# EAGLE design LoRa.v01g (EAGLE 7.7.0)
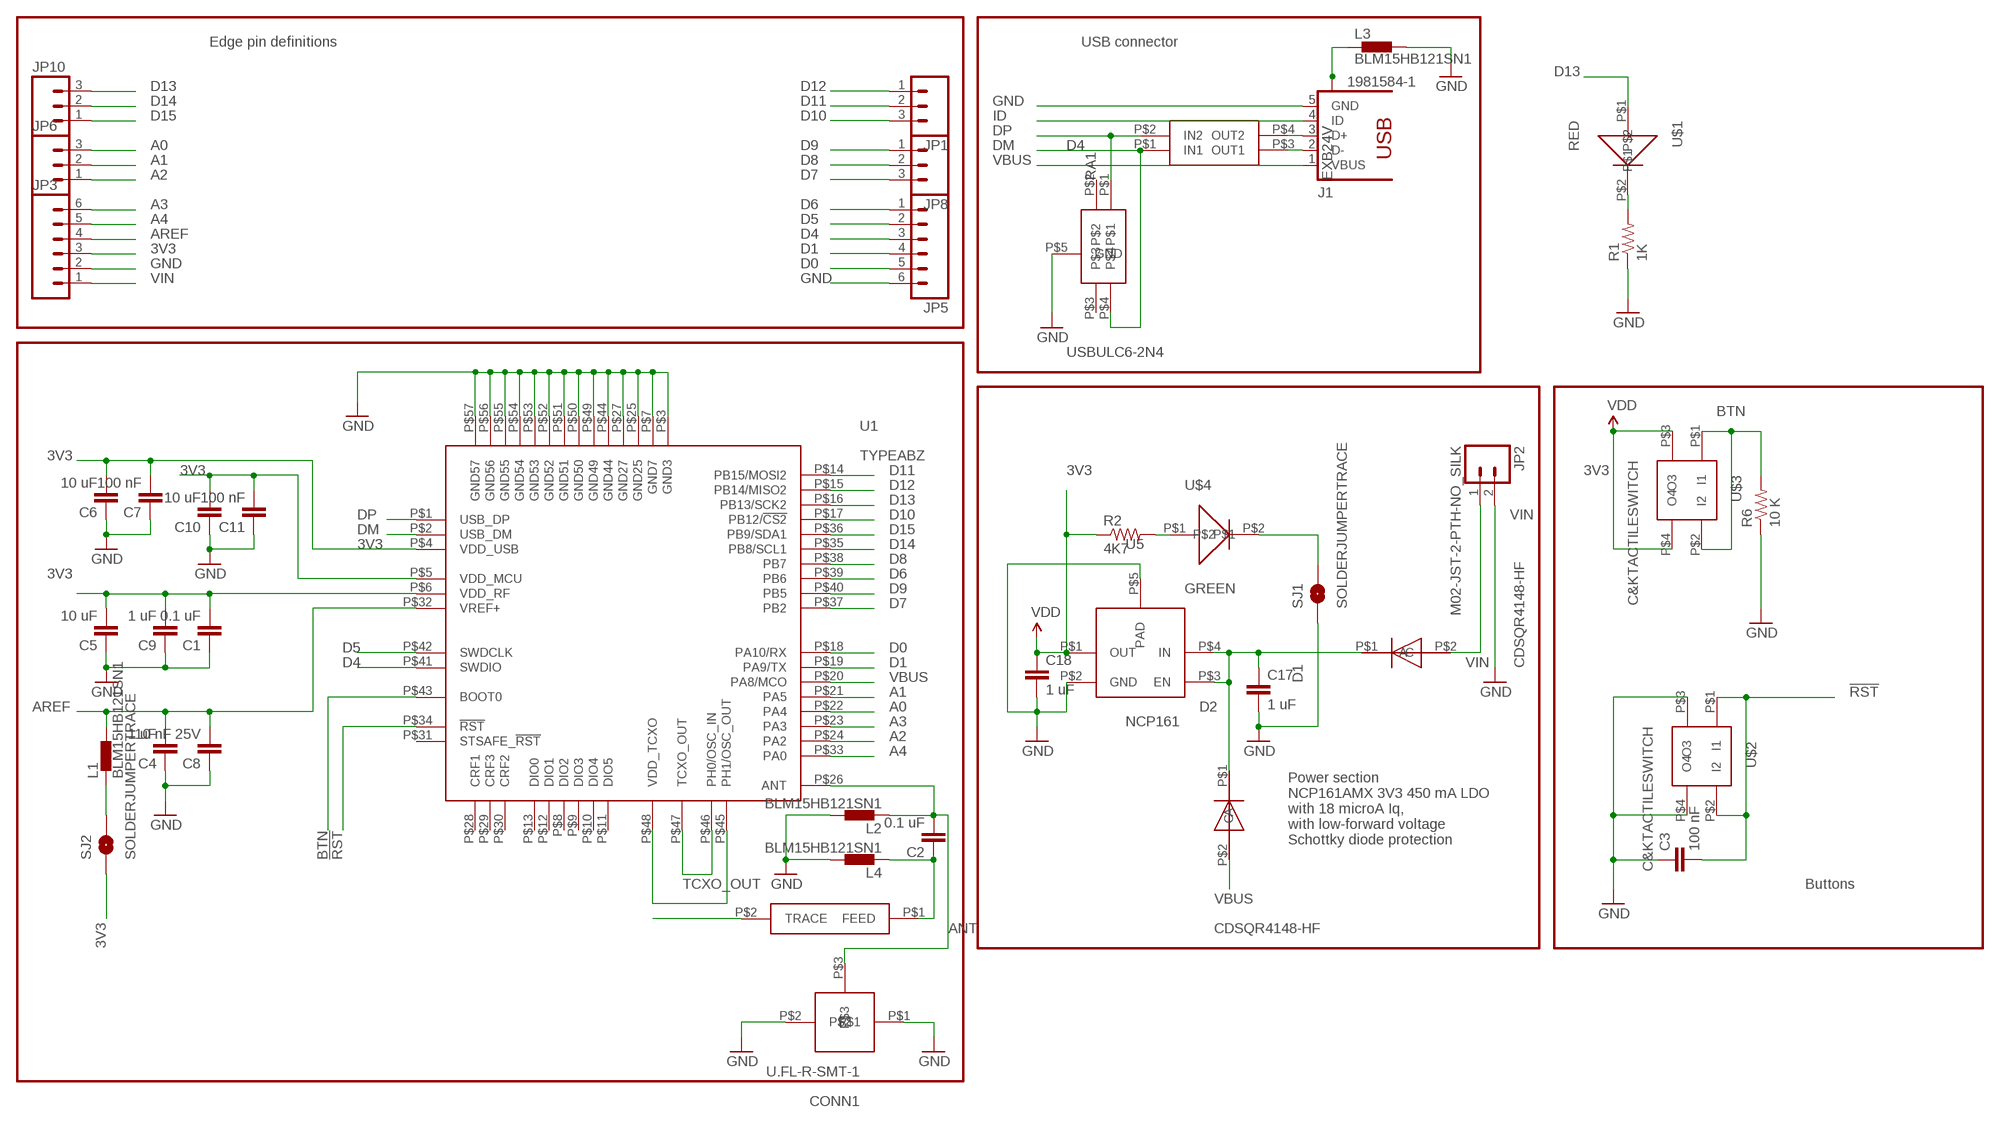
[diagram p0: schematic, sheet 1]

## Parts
C1  0.1 uF  0402CAP.KW  [0402-CAP]
C2  0.1 uF  0402CAP.KW  [0402-CAP]
C3  100 nF  0402CAP.KW  [0402-CAP]
C4  1 uF  0402CAP.KW  [0402-CAP]
C5  10 uF  0402CAP.KW  [0402-CAP]
C6  10 uF  0402CAP.KW  [0402-CAP]
C7  100 nF  0402CAP.KW  [0402-CAP]
C8  10 nF 25V  0402CAP.KW  [0402-CAP]
C9  1 uF  0402CAP.KW  [0402-CAP]
C10  10 uF  0402CAP.KW  [0402-CAP]
C11  100 nF  0402CAP.KW  [0402-CAP]
C17  1 uF  0402CAP.KW  [0402-CAP]
C18  1 uF  0402CAP.KW  [0402-CAP]
CONN1  U.FL-R-SMT-1  [U.FL-R-SMT-1]
D1  CDSQR4148-HF  [CDSQR4148-HF]
D2  CDSQR4148-HF  [CDSQR4148-HF]
D4  USBULC6-2N4  [USBULC6-2N4]
J1  1981584-1  [1981584-1]
JP1  M031X03_NO_SILK  [1X03_NO_SILK]
JP2  M02-JST-2-PTH-NO_SILK  [JST-2-PTH-NS]
JP3  M06NO_SILK  [1X06_NO_SILK]
JP5  M06NO_SILK  [1X06_NO_SILK]
JP6  M031X03_NO_SILK  [1X03_NO_SILK]
JP8  M031X03_NO_SILK  [1X03_NO_SILK]
JP10  M031X03_NO_SILK  [1X03_NO_SILK]
L1  BLM15HB121SN1  [0402]
L2  BLM15HB121SN1  [0402]
L3  BLM15HB121SN1  [0402]
L4  BLM15HB121SN1  [0402]
R1  1K  0402RES.KW  [0402-RES]
R2  4K7  0402RES.KW  [0402-RES]
R6  10 K  0402RES.KW  [0402-RES]
RA1  EXB24V  [EXB24V]
SJ1  SOLDERJUMPERTRACE  [SJ_2S-TRACE]
SJ2  SOLDERJUMPERTRACE  [SJ_2S-TRACE]
U1  TYPEABZ  [TYPEABZ]
U5  NCP161  [NCP161]
U$1  RED  0402LED  [0402LED]
U$2  C&KTACTILESWITCH  [C&KTACTILESWITCH]
U$3  C&KTACTILESWITCH  [C&KTACTILESWITCH]
U$4  GREEN  0402LED  [0402LED]
U$5  JOHANSON0900AT43A0070  [JOHANSON0900AT43A0070]

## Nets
3V3: C1.2 C5.2 C6.2 C7.2 C9.2 C10.2 C11.2 C18.1 JP3.3 R2.1 SJ2.1 U1.P$4(VDD_USB) U1.P$5(VDD_MCU) U1.P$6(VDD_RF) U5.P$1(OUT) U$3.P$3(O3) U$3.P$4(O4) ; supply symbol labelled VDD
!RST: C3.2 U1.P$34(!RST) U$2.P$1(I1) U$2.P$2(I2)
A0: JP6.3 U1.P$22(PA4)
A1: JP6.2 U1.P$21(PA5)
A2: JP6.1 U1.P$24(PA2)
A3: JP3.6 U1.P$23(PA3)
A4: JP3.5 U1.P$33(PA0)
ANT: C2.1 L4.1 U$5.P$1(FEED)
AREF: C4.2 C8.2 JP3.4 L1.2 U1.P$32(VREF+)
BTN: R6.2 U1.P$43(BOOT0) U$3.P$1(I1) U$3.P$2(I2)
D0: JP5.5 U1.P$18(PA10/RX)
D1: JP5.4 U1.P$19(PA9/TX)
D4: JP5.3 U1.P$41(SWDIO)
D5: JP5.2 U1.P$42(SWDCLK)
D6: JP5.1 U1.P$39(PB6)
D7: JP8.3 U1.P$37(PB2)
D8: JP8.2 U1.P$38(PB7)
D9: JP8.1 U1.P$40(PB5)
D10: JP1.3 U1.P$17(PB12/!CS2)
D11: JP1.2 U1.P$14(PB15/MOSI2)
D12: JP1.1 U1.P$15(PB14/MISO2)
D13: JP10.3 U1.P$16(PB13/SCK2) U$1.P$1
D14: JP10.2 U1.P$35(PB8/SCL1)
D15: JP10.1 U1.P$36(PB9/SDA1)
DM: D4.P$4 RA1.P$1(IN1) U1.P$2(USB_DM)
DP: D4.P$1 RA1.P$2(IN2) U1.P$1(USB_DP)
GND: C1.1 C3.1 C4.1 C5.1 C6.1 C7.1 C8.1 C9.1 C10.1 C11.1 C17.2 C18.2 CONN1.P$1 CONN1.P$2 D4.P$5(GND) J1.5(GND) JP2.2 JP3.2 JP5.6 L2.2 L3.2 L4.2 R1.1 R6.1 SJ1.1 U1.P$3(GND3) U1.P$7(GND7) U1.P$25(GND25) U1.P$27(GND27) U1.P$44(GND44) U1.P$49(GND49) U1.P$50(GND50) U1.P$51(GND51) U1.P$52(GND52) U1.P$53(GND53) U1.P$54(GND54) U1.P$55(GND55) U1.P$56(GND56) U1.P$57(GND57) U5.P$2(GND) U5.P$5(PAD) U$2.P$3(O3) U$2.P$4(O4)
ID: J1.4(ID)
N$1: R1.2 U$1.P$2
N$2: U$5.P$2(TRACE)
N$6: L1.1 SJ2.2
N$9: U1.P$45(PH1/OSC_OUT) U1.P$48(VDD_TCXO)
N$13: SJ1.2 U$4.P$2
N$31: J1.3(D+) RA1.P$4(OUT2)
N$32: C2.2 CONN1.P$3 L2.1 U1.P$26(ANT)
N$33: J1.2(D-) RA1.P$3(OUT1)
N$42: R2.2 U$4.P$1
N$60: C17.1 D1.P$1(C) D2.P$1(C) U5.P$3(EN) U5.P$4(IN)
TCXO_OUT: U1.P$46(PH0/OSC_IN) U1.P$47(TCXO_OUT)
USB_SHIELD: J1.S1 J1.S2 J1.S3 J1.S4 L3.1
VBUS: D2.P$2(A) J1.1(VBUS) U1.P$20(PA8/MCO)
VIN: D1.P$2(A) JP2.1 JP3.1
Unconnected: D4.P$2 D4.P$3 U1.P$8(DIO2) U1.P$9(DIO3) U1.P$10(DIO4) U1.P$11(DIO5) U1.P$12(DIO1) U1.P$13(DIO0) U1.P$28(CRF1) U1.P$29(CRF3) U1.P$30(CRF2) U1.P$31(STSAFE_!RST)

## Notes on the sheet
- Edge pin definitions | USB connector
- Power section
  NCP161AMX 3V3 450 mA LDO
  with 18 microA Iq, 
  with low-forward voltage 
  Schottky diode protection
- Buttons

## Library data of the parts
C1-C11 C17 C18 = SparkFun-Capacitors:0402CAP.KW
CONN1 = Kris:U.FL-R-SMT-1: U.FL-R-SMT-1
D1 D2 = Kris:CDSQR4148-HF: ComChip's CDSQR4148-HF high speed 150 mA Io diode
D4 = Kris:USBULC6-2N4: ST TVS diode ESD Protection USBULC6-2N4
J1 = con-usb:1981584-1: Receptacle, micro-USB, type A/B Tyco Electronics; MF: Hirose; MPN: ZX62-AB-5PA(11)
JP1 JP6 JP8 JP10 = SparkFun-Connectors:M03: Header 3 Standard 3-pin 0.1" header. Use with straight break away headers (SKU : PRT-00116), right angle break away headers (PRT-00553), swiss pins (PRT-00743), machine pins (PRT-00117), and female headers (PRT-00115). Molex polarized connector foot print use with SKU : PRT-08232 with associated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
JP2 = SparkFun-Connectors:M02: Standard 2-pin 0.1" header. Use with
JP3 JP5 = SparkFun-Connectors:M06: Header 6 Standard 6-pin 0.1" header. Use with straight break away headers (SKU : PRT-00116), right angle break away headers (PRT-00553), swiss pins (PRT-00743), machine pins (PRT-00117), and female headers (PRT-00115). Molex polarized connector foot print use with SKU : PRT-08094 with associated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
L1-L4 = inductors:BLM15H: EMIFIL (R) Chip Ferrite Bead for GHz Noise
R1 R2 R6 = SparkFun-Resistors:0402RES.KW
RA1 = Kris:EXB24V: Panasonic EXB24 22 Ohm series resistor pair
SJ1 SJ2 = SparkFun-Passives:SOLDERJUMPER: Solder Jumper
U1 = Kris:TYPEABZ: CMWX1ZZABZ-078
U5 = Kris:NCP161: NCP161 3V3 LDO voltage regulator
U$1 U$4 = Kris:0402LED: 0402led
U$2 U$3 = Kris:C&KTACTILESWITCH: C&K Tactile Switch 611-PTS810SJS250SMTR
U$5 = Kris:JOHANSON0900AT43A0070: Johanson dual wide band antenna

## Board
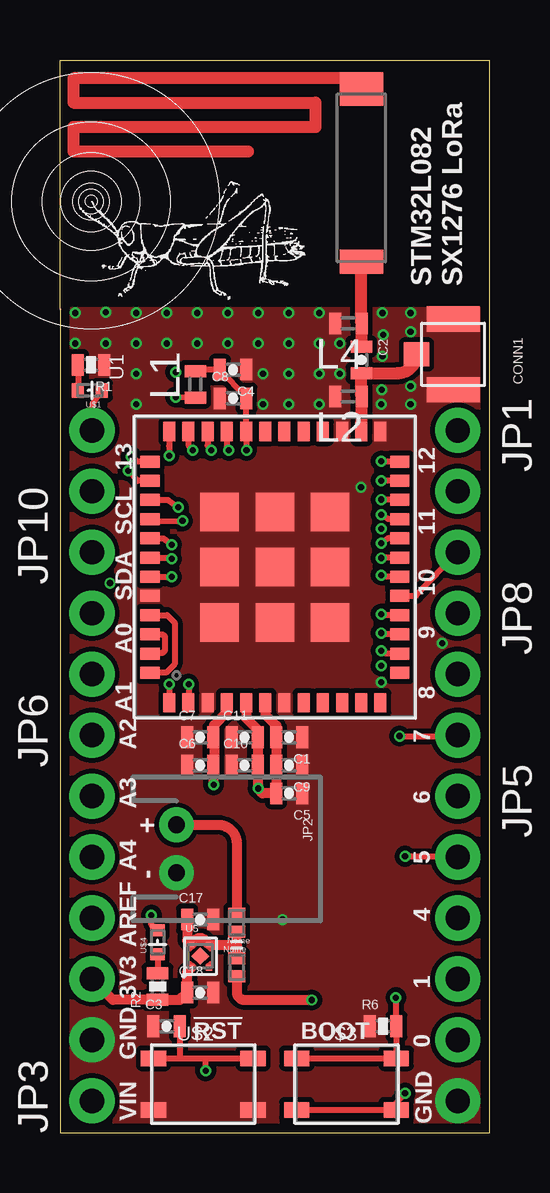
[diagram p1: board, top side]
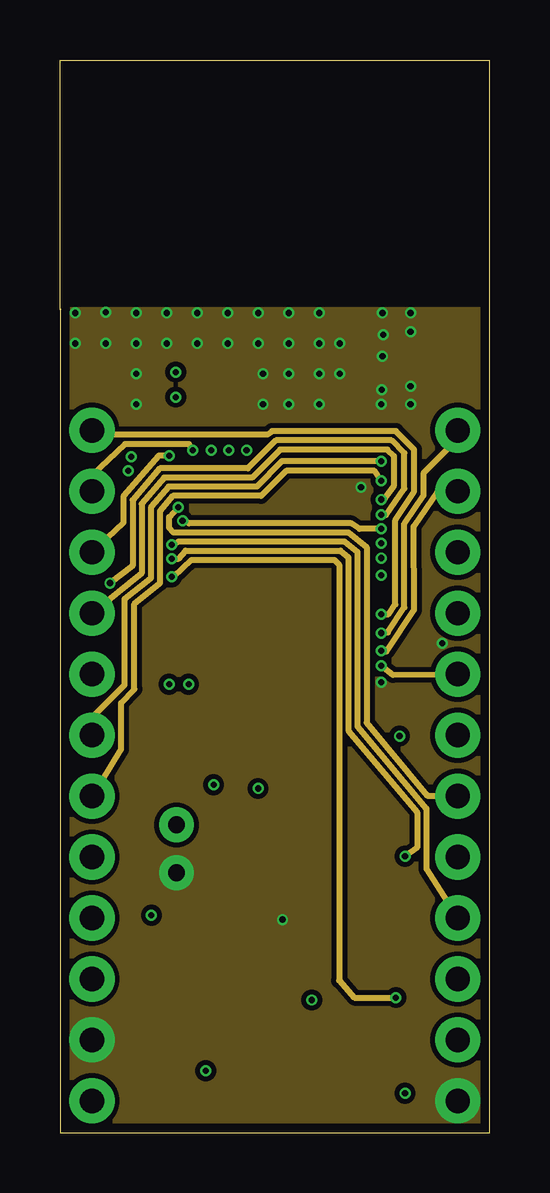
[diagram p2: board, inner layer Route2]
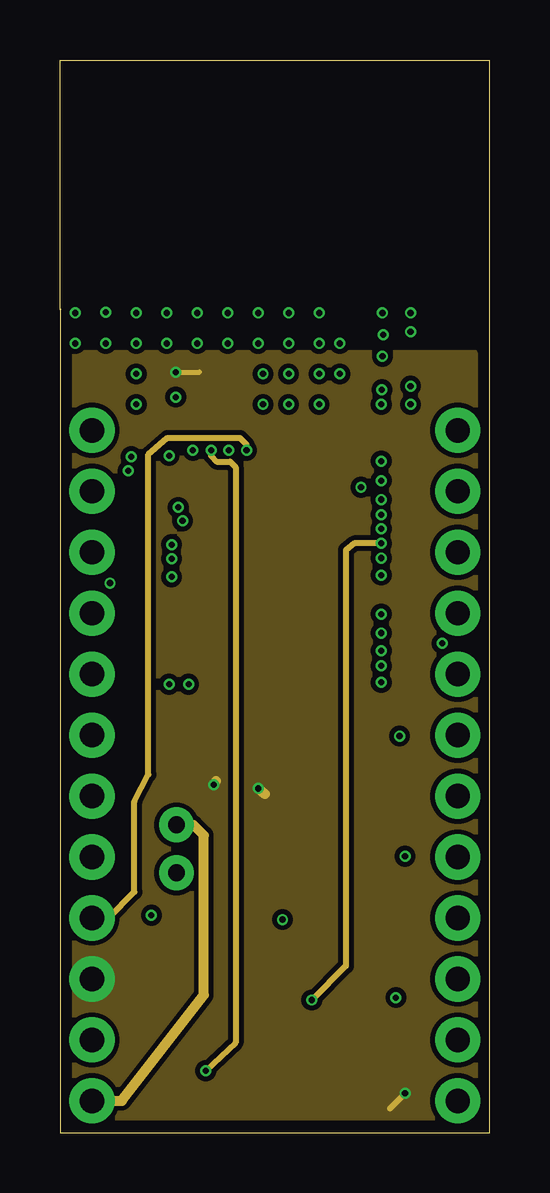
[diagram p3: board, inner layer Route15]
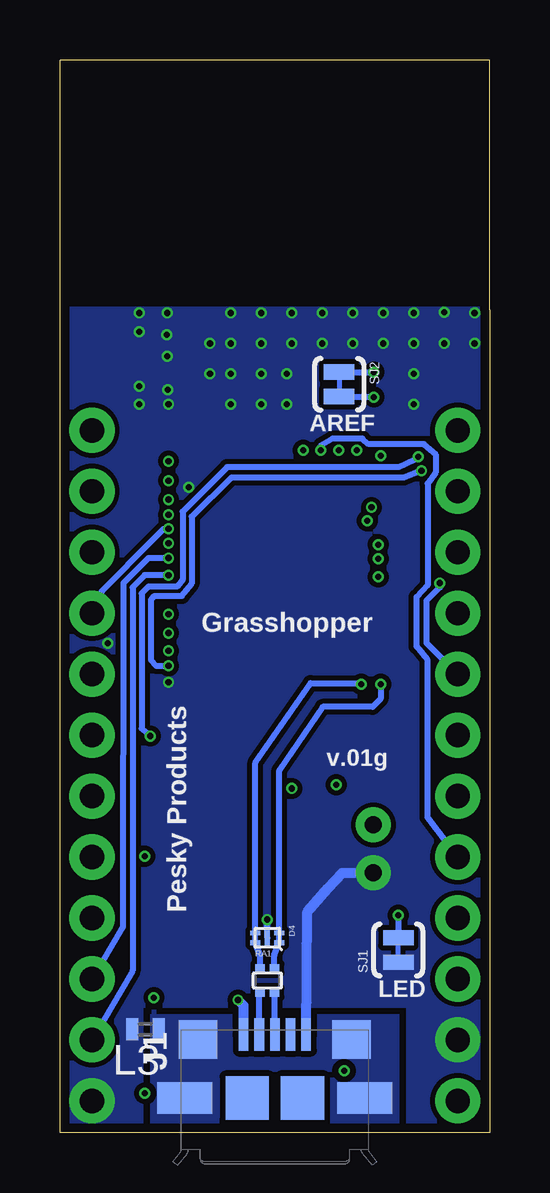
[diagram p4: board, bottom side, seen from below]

Size 17.91 x 44.7 mm. Coordinates in mm from the lower left corner, seen from the top.
Outline: 0,34.29 0,0 17.91,0 17.91,44.7 0,44.7 0,34.29
Outline: 0.03,34.31 0,34.29
Copper layers (1*2*15*16): Top 0.035559375mm / dielectric 0.17018125mm / Route2 0.01778125mm / dielectric 47mil / Route15 0.01778125mm / dielectric 0.17018125mm / Bottom 0.035559375mm
Design rules "OSHPark-4layer *": minimum track width 5mil, minimum drill 10mil, track to track 5mil, track to pad 5mil, pad to pad 5mil, via to via 5mil, smd to smd 5mil, copper to edge 15mil, drill to drill 6mil, minimum pad ring 4mil, minimum via ring 4mil, stop-mask expansion 4mil, vias tented up to drill 20mil, thermal gap 10mil

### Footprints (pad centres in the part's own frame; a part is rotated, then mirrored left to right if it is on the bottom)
0402-CAP = smd 0.5 x 0.9: 1 -0.55,0; 2 0.55,0
U.FL-R-SMT-1 = smd 1.05 x 2.2: P$1 -1.475,0; P$2 1.475,0 | smd 1 x 1.05: P$3 0,-1.525
CDSQR4148-HF = smd 0.7 x 0.5: P$1 0,0.375; P$2 0,-0.375
USBULC6-2N4 = smd 0.2 x 0.4: P$1 0.2,0.5; P$2 -0.2,0.5; P$3 -0.2,-0.5; P$4 0.2,-0.5 | smd 0.6 x 0.2: P$5 0,0
1981584-1 = smd 0.4 x 1.35: 1 -1.3,4.1; 2 -0.65,4.1; 3 0,4.1; 4 0.65,4.1; 5 1.3,4.1 | smd 1.8 x 1.8: M1 -1.15,1.45; M2 1.15,1.45 | smd 2.3 x 1.3: S1 -3.75,1.45; S2 3.75,1.45 | smd 1.6 x 1.6: S3 -3.2,3.885; S4 3.2,3.885
1X03_NO_SILK = drill 1.016 pad 1.88: 1 0,0; 2 2.54,0; 3 5.08,0
JST-2-PTH-NS = drill 0.7 pad 1.448: 1 -1,0; 2 1,0
1X06_NO_SILK = drill 1.016 pad 1.88: 1 0,0; 2 2.54,0; 3 5.08,0; 4 7.62,0; 5 10.16,0; 6 12.7,0
0402 = smd 0.5 x 0.9: 1 -0.55,0; 2 0.55,0
0402-RES = smd 0.5 x 0.9: 1 -0.55,0; 2 0.55,0
EXB24V = smd 0.4 x 0.36: P$1 -0.3,0.5; P$2 0.3,0.5; P$3 -0.3,-0.5; P$4 0.3,-0.5
SJ_2S-TRACE = smd 0.635 x 1.27: 1 -0.508,0; 2 0.508,0
TYPEABZ = smd 0.8 x 0.5: P$1 -5.65,4.4; P$2 -5.65,3.6; P$3 -5.65,2.8; P$4 -5.65,2; P$5 -5.65,1.2; P$6 -5.65,0.4; P$7 -5.65,-0.4; P$8 -5.65,-1.2; P$9 -5.65,-2; P$10 -5.65,-2.8; P$11 -5.65,-3.6; P$12 -5.65,-4.4; P$25 5.65,-4.4; P$26 5.65,-3.6; P$27 5.65,-2.8; P$28 5.65,-2; P$29 5.65,-1.2; P$30 5.65,-0.4; P$31 5.65,0.4; P$32 5.65,1.2; P$33 5.65,2; P$34 5.65,2.8; P$35 5.65,3.6; P$36 5.65,4.4 | smd 0.5 x 0.8: P$13 -4.4,-5.2; P$14 -3.6,-5.2; P$15 -2.8,-5.2; P$16 -2,-5.2; P$17 -1.2,-5.2; P$18 -0.4,-5.2; P$19 0.4,-5.2; P$20 1.2,-5.2; P$21 2,-5.2; P$22 2.8,-5.2; P$23 3.6,-5.2; P$24 4.4,-5.2; P$37 4.4,5.2; P$38 3.6,5.2; P$39 2.8,5.2; P$40 2,5.2; P$41 1.2,5.2; P$42 0.4,5.2; P$43 -0.4,5.2; P$44 -1.2,5.2; P$45 -2,5.2; P$46 -2.8,5.2; P$47 -3.6,5.2; P$48 -4.4,5.2 | smd 1.6 x 1.6: P$49 -2.3,2.3; P$50 0,2.3; P$51 2.3,2.3; P$52 -2.3,0; P$53 0,0; P$54 2.3,0; P$55 -2.3,-2.3; P$56 0,-2.3; P$57 2.3,-2.3
NCP161 = smd 0.24 x 0.24: P$1 -0.37,-0.48; P$2 0.37,-0.48; P$3 0.37,0.48; P$4 -0.37,0.48 | smd 0.52 x 0.52 rotated 45: P$5 0,0
0402LED = smd 0.5 x 0.6: P$1 -0.5,0; P$2 0.5,0
C&KTACTILESWITCH = smd 1.05 x 0.65: P$1 -2.075,1.073; P$2 2.075,1.075; P$3 -2.075,-1.075; P$4 2.075,-1.075
JOHANSON0900AT43A0070 = smd 1 x 1.8: P$1 -3.5,0 | smd 1.4 x 1.8: P$2 3.7,0

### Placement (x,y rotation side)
C1  9.55,16.48 180 top
C2  12.56,32.21 270 top
C3  4.45,4.45 0 top
C4  7.21,31.8 180 top
C5  9.55,14.15 180 top
C6  5.84,15.32 0 top
C7  5.84,16.48 0 top
C8  7.21,30.61 0 top
C9  9.55,15.32 180 top
C10  7.7,15.32 0 top
C11  7.7,16.48 0 top
C17  5.84,8.89 0 top
C18  5.84,5.84 0 top
CONN1  16.38,32.44 270 top
D1  7.37,8.76 180 top
D2  7.37,6.91 0 top
D4  9.27,8.13 270 bottom
J1  8.95,0 0 bottom
JP1  16.57,29.27 270 top
JP2  4.85,11.84 270 top
JP3  1.33,1.33 90 top
JP5  16.57,14.03 270 top
JP6  1.33,16.57 90 top
JP8  16.57,21.65 270 top
JP10  1.33,24.19 90 top
L1  5.64,31.19 90 top
L2  12.01,30.68 180 top
L3  14.35,4.32 180 bottom
L4  12.01,33.73 180 top
R1  1.3,32 180 top
R2  4.06,6.1 90 top
R6  13.46,4.45 0 top
RA1  9.27,6.35 0 bottom
SJ1  3.81,7.62 90 bottom
SJ2  6.27,31.19 270 bottom
U1  8.95,23.57 90 top
U5  5.84,7.37 0 top
U$1  1.24,30.94 180 top
U$2  5.97,2.03 0 top
U$3  11.94,2.03 0 top
U$4  4.06,7.95 90 top
U$5  12.56,39.79 90 top
U$6  [GRASSHOPPER]  0.58,34.62 0 top

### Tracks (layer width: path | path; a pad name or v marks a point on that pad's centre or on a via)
3V3  (via drill 0.25)
  Top 0.254: v14.38,1.65 13.73,0.98 U$3.P$4 U$3.P$3
  Top 0.406: U5.P$1 5.29,6.71 C18.1 5,5.55 R2.1 2.2,5.55 JP3.3 | U1.P$5 7.75,17.28 8.25,16.79 C11.2 C10.2 8.25,14.49 v8.26,14.35 8.43,14.15 C5.2 C9.2 C1.2 9.02,16.5 9.02,16.97 8.55,17.43 U1.P$6 | 6.91,17.93 U1.P$4 6.95,17.52 6.43,16.99 6.43,16.52 | v6.4,14.5 6.39,14.75 C6.2 6.43,15.35 6.43,16.52 | 6.43,16.52 C7.2
  Route15 0.203: v4.83,31.7 5.82,31.7
  Route15 0.254: v14.38,1.65 13.74,1.02
  Route15 0.406: v8.26,14.35 8.53,14.12 | v6.4,14.5 6.5,14.66
  Bottom 0.254: SJ2.1 v4.83,31.7
  pour Route15 (isolate 0.203, no thermals): 0.64,32.51 17.27,32.51 17.27,0.64 0.64,0.64
!RST  (via drill 0.25)
  Top 0.254: U$2.P$1 5,3.1 | 5,3.1 6.07,3.1 | 6.07,3.1 8.17,3.1 U$2.P$2 | C3.2 5,3.11 5,3.1 | U1.P$34 6.15,28.64 v6.3,28.45 | v6.07,2.59 6.07,3.1
  Route15 0.254: v6.3,28.45 6.3,28.22 6.53,27.96 7.09,27.96 7.32,27.74 7.32,3.76 v6.07,2.59
A0  (via drill 0.25)
  Top 0.254: U1.P$22 13.56,26.37 v13.39,26.39
  Route2 0.254: v13.39,26.39 13.54,26.44 13.92,26.98 13.92,28.19 13.64,28.47 9.17,28.47 8,27.3 4.34,27.3 3.4,26.21 3.4,23.32 JP6.3
A1  (via drill 0.25)
  Top 0.254: U1.P$21 13.67,25.57 v13.39,25.76
  Route2 0.254: v13.39,25.76 13.59,25.76 14.35,26.85 14.35,28.32 13.82,28.85 8.99,28.85 7.82,27.69 4.17,27.69 3.02,26.36 3.02,23.62 v2.08,22.91
  Bottom 0.254: v2.08,22.91 2.08,22.73 2.64,22.17 2.64,20.42 JP6.2
A2  (via drill 0.25)
  Top 0.254: U1.P$24 13.42,27.97 v13.39,27.99
  Route2 0.254: v13.39,27.99 9.25,27.99 8.2,26.92 4.52,26.92 3.79,26.06 3.79,23.11 2.69,22.25 2.69,18.67 1.33,17.31 JP6.1
A3  (via drill 0.25)
  Top 0.254: U1.P$23 13.73,27.18 v13.39,27.18
  Route2 0.254: v13.39,27.18 13.11,27.58 9.42,27.58 8.38,26.54 4.7,26.54 4.17,25.91 4.17,22.91 3.1,22.05 3.1,18.49 2.54,17.91 2.54,15.98 JP3.6
A4  (via drill 0.25)
  Top 0.254: U1.P$33 6.95,28.5 v7.04,28.45
  Bottom 0.254: v7.04,28.45 7.04,28.65 6.55,28.93 5.31,28.93 5.05,28.7 2.74,28.7 2.26,28.27 2.26,27.51 2.59,27.05 2.59,22.81 3.05,22.33 3.05,20.27 2.59,19.71 2.59,13.13 JP3.5
ANT
  Top 0.305: C2.1 | L4.1
  Top 0.508: C2.1 L4.1 | L4.1 U$5.P$1
AREF  (via drill 0.25)
  Top 0.254: L1.2 5.68,31.8 C4.2 7.76,30.62 C8.2 7.76,29.22 U1.P$32 7.77,29.02 v7.77,28.45
  Route15 0.254: JP3.4 2.02,8.95 3.1,10.05 3.1,13.82 3.68,14.94 3.68,28.27 4.47,28.96 7.49,28.96 7.77,28.68 v7.77,28.45
BTN  (via drill 0.25)
  Top 0.254: U$3.P$1 13.76,3.1 U$3.P$2 14.01,3.36 R6.2 13.99,4.46 v13.99,5.64 | U1.P$43 v4.64,23.17 4.65,23.14 v4.65,23.16
  Route2 0.254: v4.65,23.16 4.75,23.16 5.49,23.88 11.43,23.88 11.63,23.67 11.63,6.35 12.27,5.64 v13.99,5.64
D0  (via drill 0.25)
  Top 0.254: U1.P$18 13.46,23.17 v13.39,23.24
  Bottom 0.254: v13.39,23.24 14.38,23.24 14.88,22.73 14.88,6.76 JP5.5
D1  (via drill 0.25)
  Top 0.254: U1.P$19 13.46,23.97 v13.39,23.95
  Bottom 0.254: v13.39,23.95 14.22,23.95 15.27,22.91 15.29,8.59 JP5.4
D4  (via drill 0.25)
  Top 0.254: U1.P$41 4.31,24.77 v4.65,24.51
  Route2 0.254: JP5.3 15.27,11 15.27,13.51 12.39,16.94 12.39,24.21 11.86,24.64 4.93,24.64 v4.65,24.51
D5  (via drill 0.25)
  Top 0.254: U1.P$42 4.6,23.97 v4.65,23.93 | v14.38,11.53 16.54,11.53 JP5.2
  Route2 0.254: v4.65,23.93 4.95,23.93 5.23,24.26 11.68,24.26 12.01,23.98 12.01,16.76 14.88,13.36 14.88,11.89 v14.38,11.53
D6  (via drill 0.25)
  Top 0.254: U1.P$39 4.49,26.37 v4.93,26.06
  Route2 0.254: v4.93,26.06 4.55,25.65 4.55,25.22 4.72,25.02 12.01,25.02 12.78,24.41 12.78,17.09 15.33,14.03 JP5.1
D7  (via drill 0.25)
  Top 0.254: U1.P$37 3.25,27.97 v2.97,28.17 | v14.15,16.54 16.54,16.54 JP8.3
  Bottom 0.254: v2.97,28.17 3.15,28.04 3.81,27.74 10.95,27.74 12.8,25.88 12.8,23.04 13.03,22.76 14.22,22.76 14.5,22.48 14.5,16.84 v14.15,16.54
D8  (via drill 0.25)
  Top 0.254: U1.P$38 3.23,27.17 v2.85,27.58
  Route2 0.254: v13.39,19.46 13.87,19.09 JP8.2
  Bottom 0.254: v2.85,27.58 3.58,27.3 10.77,27.3 12.42,25.68 12.42,22.89 12.83,22.38 13.97,22.38 14.12,22.2 14.12,19.71 13.89,19.46 v13.39,19.46
D9  (via drill 0.25)
  Top 0.254: U1.P$40 4.03,25.5 v5.11,25.5
  Route2 0.254: v5.11,25.5 5.38,25.4 12.14,25.4 12.47,25.17 v13.39,25.17
  Bottom 0.254: JP8.1 16.18,22.55 13.99,24.77 13.59,25.17 v13.39,25.17
D10
  Top 0.254: U1.P$17 14.83,22.37 JP1.3
D11  (via drill 0.25)
  Top 0.254: U1.P$14 13.58,19.97 v13.39,20.09
  Route2 0.254: v13.39,20.09 13.61,20.07 14.76,21.79 14.73,25.27 15.73,26.73 JP1.2
D12  (via drill 0.25)
  Top 0.254: U1.P$15 13.47,20.77 v13.39,20.83
  Route2 0.254: v13.39,20.83 13.66,20.85 14.35,21.89 14.35,25.4 15.14,26.57 15.14,27.48 16.57,28.92 JP1.1
D13  (via drill 0.25)
  Top 0.254: U$1.P$1 1.35,30.38 1.35,29.29 JP10.3 | U1.P$16 13.48,21.57 v13.39,21.61
  Route2 0.254: v13.39,21.61 13.69,21.61 13.97,22.02 13.97,25.53 14.76,26.72 14.76,28.47 13.99,29.23 8.84,29.23 8.62,29.1 1.51,29.1 JP10.3
D14  (via drill 0.25)
  Top 0.254: U1.P$35 5.35,28.66 v5.54,28.45
  Route2 0.254: v5.54,28.45 5.38,28.7 2.72,28.7 1.33,27.39 JP10.2
D15  (via drill 0.25)
  Top 0.254: U1.P$36 4.55,28.62 v4.55,28.22
  Route2 0.254: v4.55,28.22 4.12,28.22 2.64,26.52 2.64,25.43 1.29,24.18 1.32,24.21 JP10.1
DM  (via drill 0.25)
  Top 0.254: v5.36,18.69 5.36,18.16 U1.P$2
  Bottom 0.254: RA1.P$1 9.57,7.4 D4.P$4 9.77,15.43 7.47,18.75 5.44,18.75 v5.36,18.69
DP  (via drill 0.25)
  Top 0.254: v4.55,18.69 U1.P$1
  Bottom 0.254: RA1.P$2 8.97,7.4 D4.P$1 8.77,15.11 6.97,17.75 4.88,17.75 4.55,18.09 v4.55,18.69
GND  (via drill 0.25)
  Bottom 0.254: D4.P$5 v9.27,8.89
  Bottom 0.406: J1.5 7.6,9.21 6.73,10.21 6.16,10.84 JP2.2
  other vias: 12.54,26.9 13.39,30.35 11.66,32.89 11.66,31.62 10.79,31.62 1.91,34.19 3.17,34.16 4.45,34.16 5.71,34.16 13.44,34.16 10.79,34.16 9.53,34.16 8.26,34.16 14.61,34.16 0.64,34.16 10.79,30.35 13.44,32.36 13.41,30.96 10.79,32.89 6.99,34.16 14.61,33.38 14.61,31.11 14.61,30.35 0.64,32.89 1.91,32.89 3.17,32.89 4.45,32.89 5.71,32.89 6.99,32.89 8.26,32.89 9.53,32.89 9.53,31.62 8.46,31.62 8.46,30.35 9.53,30.35 3.17,31.62 3.17,30.35 13.39,18.77 13.46,33.25 15.93,20.4
  pour Top (isolate 0.203, no thermals): 0,34.29 17.91,34.29 17.91,0 0,0
  pour Route2 (isolate 0.203, no thermals): 0,34.29 17.91,34.29 17.91,0 0,0
  pour Bottom (isolate 0.203, no thermals): 3.37,0 0,0 0,34.29 17.91,34.29 17.91,0 14.54,0 14.54,5.33 3.37,5.33
N$1
  Top 0.254: R1.2 0.75,31.22 U$1.P$2
N$4
  Top 0.508: 11.71,43.94 0.56,43.94 0.56,42.93
N$5
  Top 0.508: 0.56,42.93 10.64,42.93 10.64,41.91 0.56,41.91 0.56,40.89 7.82,40.89
N$6  (via drill 0.25)
  Top 0.254: L1.1 5.55,30.64 v4.83,30.66
  Bottom 0.203: 5.82,30.66 SJ2.2
  Bottom 0.254: v4.83,30.66 5.82,30.66
N$9
  Top 0.254: U1.P$45 4.46,21.57 4.78,21.26 4.78,19.53 4.42,19.18 U1.P$48
N$13  (via drill 0.25)
  Top 0.254: U$4.P$2 3.81,8.68 v3.81,9.07
  Bottom 0.254: v3.81,9.07 SJ1.2
N$31
  Bottom 0.254: J1.3 8.95,5.83 RA1.P$4
N$32
  Top 0.254: U1.P$26
  Top 0.305: U1.P$26 12.56,29.22 | L2.1
  Top 0.508: 12.56,29.22 L2.1 | L2.1 C2.2 14.05,31.66 arc90 CONN1.P$3
N$33
  Bottom 0.254: J1.2 9.6,5.82 RA1.P$3
N$42
  Top 0.254: U$4.P$1 R2.2
N$60
  Top 0.406: D2.P$1 7.37,7.8 | 7.37,7.8 D1.P$1 | 7.37,7.8 7.32,7.85 U5.P$3 5.94,8.1 5.73,8.1 U5.P$4 5.29,8.03 C17.1
TCXO_OUT
  Top 0.254: U1.P$46 4.27,20.77 4.37,20.68 4.37,20.09 4.27,19.99 3.77,19.99 U1.P$47
USB_SHIELD
  pour Bottom (isolate 0.254, rank 3, no thermals): 3.87,0 3.87,5.21 14.03,5.21 14.03,0
VBUS  (via drill 0.25)
  Top 0.254: U1.P$20 13.67,24.77 v13.39,24.56
  Top 0.406: v10.49,5.54 7.7,5.54 arc-90 7.37,5.87 D2.P$2
  Route15 0.254: 10.46,5.56 v10.49,5.54 11.91,6.96 11.91,24.28 12.27,24.56 v13.39,24.56
  Bottom 0.406: J1.1 10.25,5.3 v10.49,5.54
VIN
  Top 0.406: JP2.1 6.59,12.84 arc-90 7.37,12.06 D1.P$2
  Route15 0.406: JP3.1 2.58,1.33 5.99,5.74 5.99,12.39 5.55,12.84 JP2.1

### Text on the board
tPlace: STM32L082 / SX1276 LoRa | 13 | 12 | SCL | 11 | SDA | 10 | 9 | A0 | A1 | 8 | A2 | 7 | A3 | 6 | + | A4 | - | 5 | 4 | AREF | 3V3 | 1 | !RST | BOOT | 0 | GND | VIN | GND
bPlace: AREF | Grasshopper | Pesky Products | v.01g | LED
